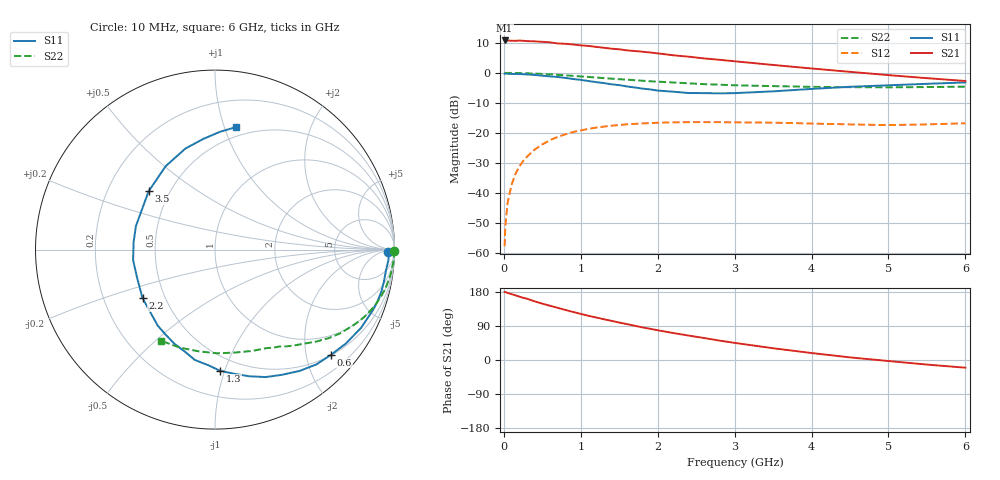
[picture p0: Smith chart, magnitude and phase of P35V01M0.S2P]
! SIEMENS Small Signal Semiconductors
! BFP181
! Si NPN RF Bipolar Junction Transistor in SOT143
! VCE = 5 V  IC = 1 mA
! Common Emitter S-Parameters:  March  1996
# GHz  S  MA  R  50
!  f  S11  S21  S12  S22
! GHz  MAG  ANG  MAG  ANG  MAG  ANG  MAG  ANG
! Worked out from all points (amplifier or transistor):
!   36 points, 10 MHz to 6 GHz, reference 50 ohm
!   highest |S21| = 10.8 dB at 10 MHz (marker M1)
!   |S21| within 3 dB of that: start of sweep to 1.515 GHz
!   unconditionally stable (mu >= 1): 3.171 GHz to end of sweep
!   at 250 MHz: K = 0.08, MSG = 20.0 dB, |S12| = -29.4 dB
!   at 1.4 GHz: K = 0.49, MSG = 12.8 dB, |S12| = -17.6 dB
!   at 6 GHz: K = 1.27, MAG = 3.9 dB, |S12| = -16.8 dB
!   lowest NFmin = 1.30 dB at 450 MHz
!   S11 on the Smith chart (normalised r, x): 10 MHz: 48, -19; 600 MHz: 0.51, -2.51; 1.3 GHz: 0.39, -0.96; 2.2 GHz: 0.37, -0.26; 3.5 GHz: 0.38, +0.33; 6 GHz: 0.42, +1.10
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0.01  0.9647 -0.8  3.464 179.6  0.0013 85.2  0.9981 -0.3
0.02  0.9682 -1.5  3.442 179.4  0.0029 83.6  0.9978 -0.6
0.05  0.9682 -3.4  3.45 176.9  0.007 91.1  0.9968 -1.7
0.1  0.9595 -7.1  3.431 173.8  0.0136 85.8  0.9978 -3.3
0.15  0.9577 -10.8  3.414 170.7  0.0206 82.6  0.9934 -5.0
0.2  0.956 -14.3  3.45 167.4  0.0274 81.0  0.9914 -6.6
0.3  0.9421 -21.0  3.38 161.8  0.0401 75.6  0.983 -10.0
0.4  0.9231 -28.2  3.348 154.9  0.0528 71.5  0.9728 -13.2
0.6  0.8731 -42.1  3.224 143.1  0.0759 62.0  0.9436 -19.3
0.8  0.8241 -55.1  3.047 132.1  0.0946 54.3  0.9099 -24.6
1.1  0.7313 -74.8  2.811 116.6  0.1168 43.5  0.8531 -31.8
1.3  0.6758 -87.6  2.617 107.6  0.1273 37.2  0.8178 -36.1
1.5  0.6249 -100.4  2.467 98.8  0.1353 32.1  0.7836 -39.7
1.8  0.5472 -120.4  2.252 86.1  0.144 25.3  0.7399 -44.5
2.2  0.486 -146.2  1.964 71.3  0.1499 17.4  0.6909 -50.7
2.4  0.4616 -160.1  1.861 64.5  0.151 14.1  0.6701 -53.6
2.8  0.4554 174.6  1.652 51.3  0.1509 8.9  0.6359 -59.2
3.5  0.4923 138.7  1.354 31.0  0.1482 2.3  0.6017 -69.7
4  0.5402 120.5  1.183 18.4  0.1432 -0.4  0.5848 -78.7
4.5  0.5866 106.3  1.04 6.9  0.1385 -2.1  0.578 -88.7
5.5  0.6568 87.6  0.816 -12.1  0.1385 0.8  0.58 -109.5
6  0.6929 80.2  0.732 -20.3  0.1448 1.6  0.5899 -120.4
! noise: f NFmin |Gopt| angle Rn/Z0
0.45  1.3  0.7  18  0.5
0.9  1.4  0.6  39  0.52
1.8  1.85  0.4  81  0.47
